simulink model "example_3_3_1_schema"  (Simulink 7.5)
settings: Solver=ode45  StartTime=0.0  StopTime=50  MaxStep=0.001  RelTol=1e-3
undefined symbols (not defined in the file or in its folder): a, b
libraries: simulink x2

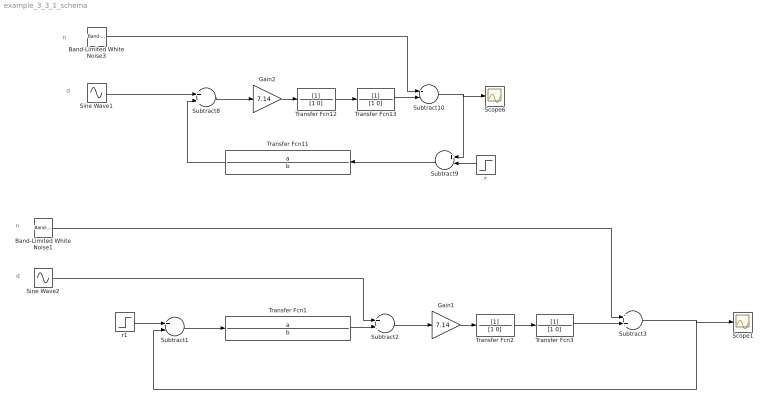
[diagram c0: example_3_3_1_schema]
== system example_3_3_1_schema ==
  note: n
  note: d
  note: d
  note: n
  Band-Limited White Noise1 : simulink/Sources/Band-Limited White Noise  SystemSampleTime=-1  Cov=[0.00001]  Ts=0.010  seed=[10]
  Band-Limited White Noise3 : simulink/Sources/Band-Limited White Noise  SystemSampleTime=-1  Cov=[0.00001]  Ts=0.010  seed=[10]
  Gain1 : Gain  Gain=7.14  ParameterDataType=sfix(16)  ParameterScaling=2^0  OutDataType=sfix(16)  OutScaling=2^0
  Gain2 : Gain  Gain=7.14  ParameterDataType=sfix(16)  ParameterScaling=2^0  OutDataType=sfix(16)  OutScaling=2^0
  Scope1 : Scope
  Scope6 : Scope
  Sine Wave1 : Sin  Amplitude=0.1  Bias=0  Frequency=100  Phase=0  Samples=10  SampleTime=0
  Sine Wave2 : Sin  Amplitude=0.1  Bias=0  Frequency=100  Phase=0  Samples=10  SampleTime=0
  Subtract1 : Sum  Inputs=+-  OutDataType=sfix(16)  OutScaling=2^-10
  Subtract10 : Sum  Inputs=--  OutDataType=sfix(16)  OutScaling=2^-10
  Subtract2 : Sum  OutDataType=sfix(16)  OutScaling=2^-10
  Subtract3 : Sum  OutDataType=sfix(16)  OutScaling=2^-10
  Subtract8 : Sum  OutDataType=sfix(16)  OutScaling=2^-10
  Subtract9 : Sum  Inputs=+-  OutDataType=sfix(16)  OutScaling=2^-10
  Transfer Fcn1 : TransferFcn  Numerator=a  Denominator=b
  Transfer Fcn11 : TransferFcn  Numerator=a  Denominator=b
  Transfer Fcn{2..3,12..13} (4 alike) : TransferFcn  Denominator=[1 0]
  r : Step  Time=0  SampleTime=0
  r1 : Step  Time=0  SampleTime=0
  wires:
  Transfer Fcn12/1 -> Transfer Fcn13/1
  Subtract8/1 -> Gain2/1
  Transfer Fcn13/1 -> Subtract10/2
  Transfer Fcn11/1 -> Subtract8/2
  Band-Limited White Noise3/1 -> Subtract10/1
  Sine Wave1/1 -> Subtract8/1
  Subtract9/1 -> Transfer Fcn11/1
  Subtract10/1 -> Scope6/1, Subtract9/1
  r/1 -> Subtract9/2
  Gain2/1 -> Transfer Fcn12/1
  r1/1 -> Subtract1/1
  Subtract1/1 -> Transfer Fcn1/1
  Transfer Fcn1/1 -> Subtract2/2
  Sine Wave2/1 -> Subtract2/1
  Transfer Fcn2/1 -> Transfer Fcn3/1
  Subtract2/1 -> Gain1/1
  Transfer Fcn3/1 -> Subtract3/2
  Gain1/1 -> Transfer Fcn2/1
  Band-Limited White Noise1/1 -> Subtract3/1
  Subtract3/1 -> Subtract1/2, Scope1/1
